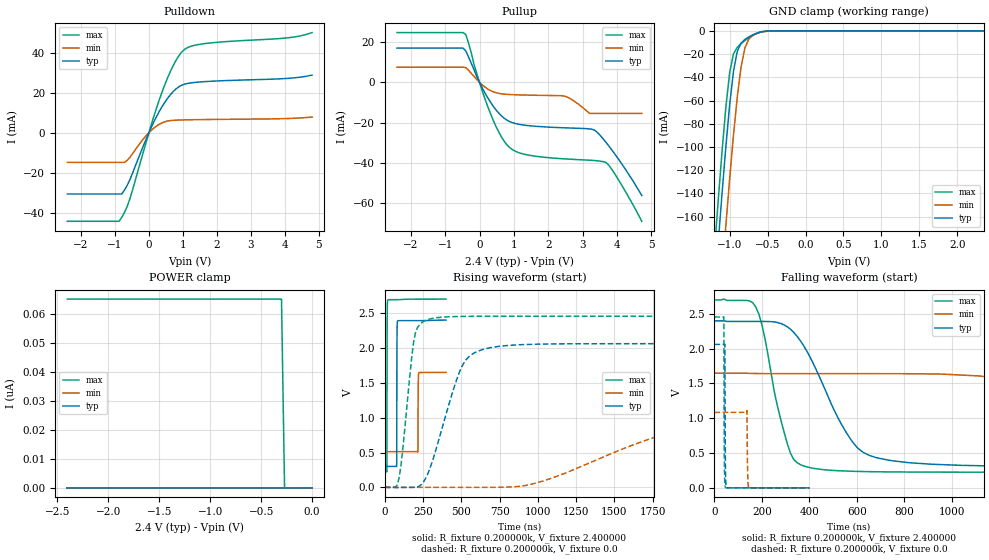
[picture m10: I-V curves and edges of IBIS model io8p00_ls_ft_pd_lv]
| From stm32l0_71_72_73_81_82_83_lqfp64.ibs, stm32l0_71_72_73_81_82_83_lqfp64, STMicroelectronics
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|   Model io8p00_ls_ft_pd_lv
[Model]  io8p00_ls_ft_pd_lv
Model_type I/O
Polarity   Non-Inverting
Enable   Active-Low
Vinl =   0.720000V
Vinh =   1.680000V
Vmeas =  1.200000V
Cref =   50.000000pF
Rref =   100.000000M
Vref =   0.0V
C_comp   4.521100pF   4.438000pF   4.578000pF
[Temperature Range]   25.000000   0.105000k   -40.000000
[Pullup Reference]   2.400000V   1.650000V   2.700000V
[Pulldown Reference]   0.0V   0.0V   0.0V
[POWER Clamp Reference]   2.400000V   1.650000V   2.700000V
[GND Clamp Reference]   0.0V   0.0V   0.0V
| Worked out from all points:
|   slope of the pulldown table from 0 to 0.36 V, typ, clamps not added: 29.5 ohm
|   slope of the pullup table from 0 to 0.36 V, typ, clamps not added: 33.2 ohm
|   GND clamp passes 1 mA (typ) near -0.59 V on its own axis
|   rising waveform, R_fixture 0.200000k, V_fixture 2.400000: 20-80 % time 1.16ns typ, 1.16ns min, 1.15ns max; typ from 0.301 V to 2.4 V
|   rising waveform, R_fixture 0.200000k, V_fixture 0.0: 20-80 % time 171ns typ, 825ns min, 66.9ns max; typ from 0 V to 2.06 V
|   falling waveform, R_fixture 0.200000k, V_fixture 2.400000: 20-80 % time 183ns typ, 739ns min, 91.1ns max; typ from 2.4 V to 0.301 V
|   falling waveform, R_fixture 0.200000k, V_fixture 0.0: 20-80 % time 1.73ns typ, 2.33ns min, 1.51ns max; typ from 2.06 V to 0 V
[Pulldown]
|Voltage   I(typ)   I(min)   I(max)
-2.4V     -30.64mA   -14.84mA   -44.29mA
-880mV    -30.64mA   -14.84mA   -44.29mA
-800mV    -30.64mA   -14.84mA   -42.37mA
-560mV    -23.52mA   -12.34mA   -33.09mA
0V        -765.1nA   -61.09nA   -2.527uA
400mV     13.38mA    4.998mA    20.91mA
720mV     20.62mA    6.178mA    33.69mA
880mV     22.92mA    6.306mA    38.42mA
1.04V     24.19mA    6.384mA    41.49mA
1.6V      25.46mA    6.543mA    44.41mA
4.08V     27.12mA    7.07mA     47.39mA
4.8V      28.77mA    7.815mA    50.01mA
[Pullup]
|Voltage   I(typ)   I(min)   I(max)
-2.4V     17.06mA    7.581mA    24.76mA
-400mV    15.68mA    7.363mA    23.82mA
-80mV     2.912mA    1.472mA    4.444mA
240mV     -7.653mA   -3.251mA   -12mA
560mV     -15.22mA   -5.43mA    -24.63mA
800mV     -18.73mA   -5.908mA   -31mA
1.28V     -21.13mA   -6.236mA   -35.54mA
2.48V     -22.51mA   -6.819mA   -37.93mA
3.2V      -23.05mA   -15.37mA   -38.57mA
3.36V     -23.83mA   -15.37mA   -38.77mA
3.76V     -31.49mA   -15.37mA   -41.07mA
4.72V     -56.1mA    -15.37mA   -68.9mA
[GND_clamp]
|Voltage   I(typ)   I(min)   I(max)
-2.4V     -1.379A    -1.445A    -1.35A
-1.2V     -225.9mA   -297.5mA   -189.2mA
-1.15V    -182mA     -253.1mA   -145.3mA
-1.1V     -139.6mA   -209.7mA   -103.5mA
-1.05V    -99.62mA   -167.6mA   -65.7mA
-1V       -63.68mA   -127.3mA   -35.9mA
-950mV    -35mA      -89.93mA   -19.88mA
-900mV    -17.68mA   -57.02mA   -14.13mA
-850mV    -10.5mA    -31.19mA   -11.01mA
-750mV    -5.3mA     -7.337mA   -6.005mA
-450mV    -43.41uA   -101.2uA   -21.28uA
2.35V     52.68uA    50.02uA    36.83uA
[POWER_clamp]
|Voltage   I(typ)   I(min)   I(max)
-2.4V     0A         0A         65.17nA
-300mV    0A         0A         65.17nA
-270mV    0A         0A         0A
0V        0A         0A         0A
[Ramp]
| variable   typ   min   max
dV/dt_r  0.63713/0.30048u   0.18750/0.80986u   1.01518/0.14382u
dV/dt_f  0.74040/0.32437u   0.19470/0.84980u   1.11768/0.16285u
R_load = 50.000000
[Rising Waveform]
R_fixture= 0.200000k
V_fixture= 2.400000
V_fixture_min= 1.650000
V_fixture_max= 2.700000
|time   V(typ)   V(min)   V(max)
0s        300.9mV    513mV      224.8mV
13.61ns   300.9mV    513mV      223.9mV
15.62ns   300.9mV    513mV      2.366V
19.22ns   300.9mV    513mV      2.686V
77.68ns   304.5mV    513mV      2.691V
79.68ns   2.087V     513mV      2.691V
82.88ns   2.383V     513mV      2.691V
215.8ns   2.391V     508.5mV    2.699V
222.2ns   2.391V     1.643V     2.699V
400ns     2.398V     1.647V     2.699V
[Rising Waveform]
R_fixture= 0.200000k
V_fixture= 0.0
V_fixture_min= 0.0
V_fixture_max= 0.0
|time   V(typ)   V(min)   V(max)
0s        17.38uV    2.739uV    39.86uV
93.43ns   -108.2uV   2.739uV    134.5mV
200.2ns   1.7mV      2.739uV    2.216V
280.3ns   190.8mV    -23.17uV   2.404V
373.7ns   844.3mV    -23.32uV   2.44V
533.9ns   1.837V     6.235uV    2.451V
894.2ns   2.046V     18.68mV    2.453V
1.975us   2.06V      847.2mV    2.453V
2.803us   2.06V      1.049V     2.453V
13.33us   2.06V      1.083V     2.453V
[Falling Waveform]
R_fixture= 0.200000k
V_fixture= 2.400000
V_fixture_min= 1.650000
V_fixture_max= 2.700000
|time   V(typ)   V(min)   V(max)
0s        2.398V     1.647V     2.699V
173.5ns   2.389V     1.642V     2.601V
320.3ns   2.277V     1.64V      496.2mV
520.5ns   1.002V     1.64V      246mV
627.3ns   508.1mV    1.64V      234.3mV
814.1ns   363mV      1.639V     227.4mV
1.348us   307.7mV    1.497V     224.8mV
2.229us   301.1mV    719.5mV    224.8mV
3.016us   300.9mV    555mV      224.8mV
13.33us   300.9mV    513mV      224.8mV
[Falling Waveform]
R_fixture= 0.200000k
V_fixture= 0.0
V_fixture_min= 0.0
V_fixture_max= 0.0
|time   V(typ)   V(min)   V(max)
0s        2.06V      1.083V     2.453V
39.24ns   2.06V      1.083V     2.456V
41.64ns   2.06V      1.083V     367.4mV
43.64ns   2.062V     1.083V     57.94mV
45.65ns   496.9mV    1.083V     9.856mV
51.25ns   4.457mV    1.083V     1.047mV
136.5ns   51.4uV     1.109V     139.1uV
140.1ns   49.04uV    153.4mV    138.7uV
145.3ns   47.31uV    2.961mV    138.3uV
400ns     17.38uV    2.739uV    39.86uV
